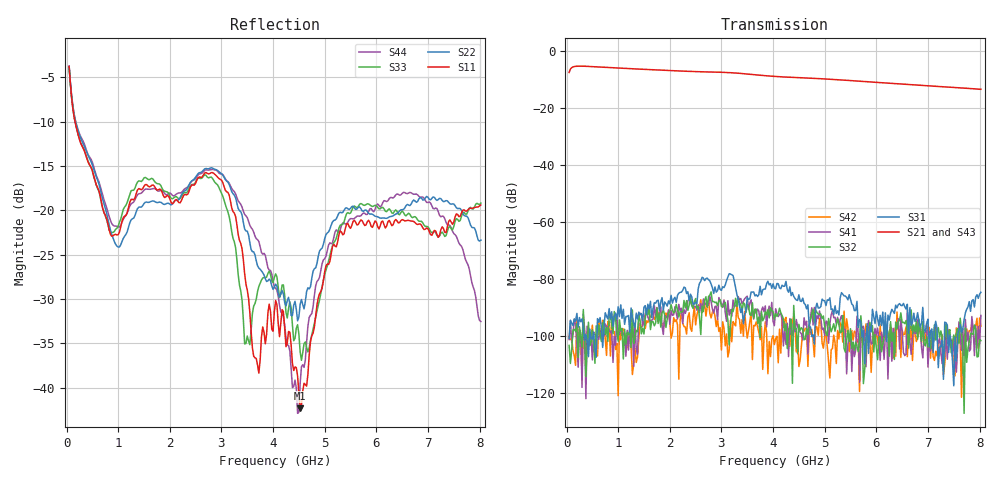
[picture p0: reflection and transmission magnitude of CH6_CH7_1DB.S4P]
!Agilent Technologies,E5071C,MY46316741,A.11.02
!Date: Mon Jun 01 10:33:44 2026
!Data & Calibration Information:
!1:CH6 INPUT 2:CH6 OUTPUT 3:CH7 INPUT 4:CH7 OUTPUT
!Freq	S11:SOLT4(ON)	S12:SOLT4(ON)	S13:SOLT4(ON)	S14:SOLT4(ON)
!	S21:SOLT4(ON)	S22:SOLT4(ON)	S23:SOLT4(ON)	S24:SOLT4(ON)
!	S31:SOLT4(ON)	S32:SOLT4(ON)	S33:SOLT4(ON)	S34:SOLT4(ON)
!	S41:SOLT4(ON)	S42:SOLT4(ON)	S43:SOLT4(ON)	S44:SOLT4(ON)
!PortZ  Port1:50+j0  Port2:50+j0  Port3:50+j0  Port4:50+j0
!Above PortZ is port z conversion or system Z0 setting when saving the data.
!When reading, reference impedance value at option line is always used.
# Hz S dB R 50
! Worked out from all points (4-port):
!   320 points, 50 MHz to 8.025 GHz, reference 50 ohm
!   strongest paths, dB at 50 MHz, 2.05 GHz, 4.05 GHz, 6.05 GHz, 8.025 GHz:
!     S21: -7.4, -6.8, -8.8, -10.9, -13.3
!     S43: -7.4, -6.7, -8.9, -11.0, -13.4
!     S31: -101.0, -88.5, -83.5, -96.5, -84.7
!     S32: -103.4, -91.0, -92.2, -100.7, -101.7
!     S41: -101.4, -92.9, -90.5, -100.9, -92.9
!     S42: -100.2, -99.1, -101.0, -105.2, -96.7
!   lowest |S11| = -42.3 dB at 4.525 GHz (marker M1), VSWR 1.02, Z = 49.9 - j0.755 ohm
!   |S11| at or under -10 dB: 164.4 MHz to end of sweep
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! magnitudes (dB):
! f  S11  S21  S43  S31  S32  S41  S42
! 50 MHz  -3.8  -7.4  -7.4  -101.0  -103.4  -101.4  -100.2
! 975 MHz  -22.8  -5.9  -5.9  -94.3  -98.7  -93.0  -102.7
! 3 GHz  -16.6  -7.3  -7.3  -84.0  -89.8  -88.7  -105.0
! 3.45 GHz  -27.2  -7.9  -7.9  -92.6  -89.0  -87.0  -91.4
! 4.525 GHz  -42.3  -9.3  -9.3  -87.8  -98.1  -98.8  -108.4
! 6.4 GHz  -21.2  -11.4  -11.5  -90.2  -97.6  -96.8  -91.7
! 8.025 GHz  -19.4  -13.3  -13.4  -84.7  -101.7  -92.9  -96.7
